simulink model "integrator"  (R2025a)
settings: Solver=ode45  StartTime=0.0  StopTime=0.1  MaxStep=1e-4  RelTol=1e-4  EnableMultiTasking=on
undefined symbols (not defined in the file): DiscIntNeverNeededParam

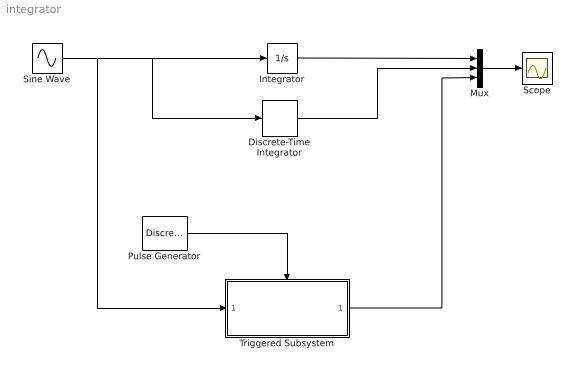
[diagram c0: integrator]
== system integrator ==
  Discrete-Time Integrator : DiscreteIntegrator  IntegratorMethod=Integration: Backward Euler  SampleTime=0.001  ICPrevOutput=DiscIntNeverNeededParam  ICPrevScaledInput=DiscIntNeverNeededParam
  Integrator : Integrator
  Mux : Mux  Inputs=3
  Pulse Generator : DiscretePulseGenerator  PulseType=Time based  Period=0.001  PulseWidth=50
  Scope : Scope
  Sine Wave : Sin  Frequency=2*pi*5  SampleTime=0
  Triggered Subsystem : Subsystem  TreatAsAtomicUnit=on
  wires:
  Sine Wave/1 -> Triggered Subsystem/1(In1), Discrete-Time Integrator/1, Integrator/1
  Integrator/1 -> Mux/1
  Mux/1 -> Scope/1
  Triggered Subsystem/1(Out1) -> Mux/3
  Pulse Generator/1 -> Triggered Subsystem/Trigger
  Discrete-Time Integrator/1 -> Mux/2

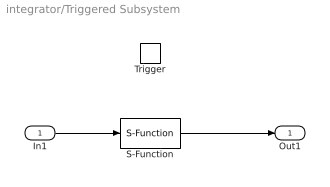
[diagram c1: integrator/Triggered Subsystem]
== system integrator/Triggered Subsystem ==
  In1 : Inport
  Trigger : TriggerPort  VariantControl=(inherit)
  S-Function : S-Function  FunctionName=controller  SFunctionDeploymentMode=off  EnableBusSupport=off
  Out1 : Outport
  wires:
  In1/1 -> S-Function/1
  S-Function/1 -> Out1/1
